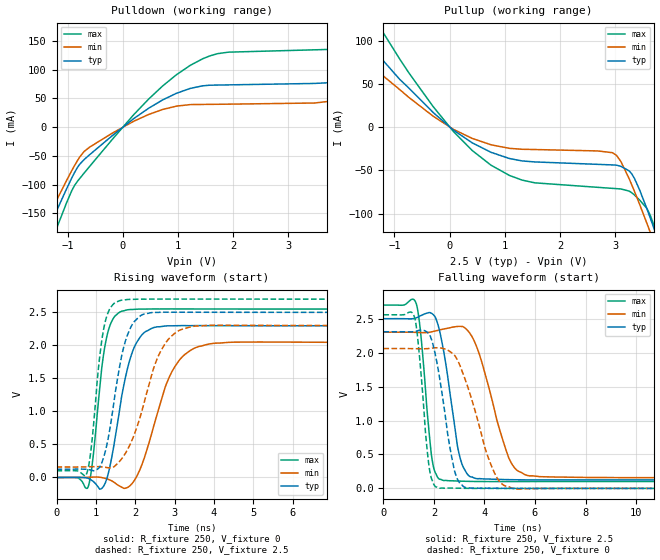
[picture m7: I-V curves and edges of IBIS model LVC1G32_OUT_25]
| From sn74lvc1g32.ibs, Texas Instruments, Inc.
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[Model]   LVC1G32_OUT_25
Model_type  Output
Vref =   0.0
Rref =   500
Cref =   30p
Vmeas =   1.25
| variable   typ   min   max
C_comp   7.81pF   3.37pF   14.37pF
| C_pullup   6.28pF   3.37pF   8.33pF
| C_pulldown   9.34pF   4.59pF   14.37pF
[Temperature Range]   40   100   -40
| Ambient temperature   25   85   -40
[Voltage range]   2.5   2.3   2.7
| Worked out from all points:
|   slope of the pulldown table from 0 to 0.375 V, typ, clamps not added: 13.9 ohm
|   slope of the pullup table from 0 to 0.375 V, typ, clamps not added: 22 ohm
|   rising waveform, R_fixture 250, V_fixture 0: 20-80 % time 442ps typ, 674ps min, 282ps max; typ from 0 V to 2.3 V
|   rising waveform, R_fixture 250, V_fixture 2.5: 20-80 % time 416ps typ, 679ps min, 265ps max; typ from 0.125 V to 2.5 V
|   falling waveform, R_fixture 250, V_fixture 2.5: 20-80 % time 561ps typ, 950ps min, 361ps max; typ from 2.5 V to 0.125 V
|   falling waveform, R_fixture 250, V_fixture 0: 20-80 % time 581ps typ, 997ps min, 347ps max; typ from 2.31 V to 0 V
[Pulldown]
| LVC1G32_OUT_25
|   Voltage   I(typ)   I(min)   I(max)
-5V       -964.5mA   -872.8mA   -1.115A
-1.565V   -226.1mA   -199.4mA   -269.6mA
-1.175V   -140.9mA   -122.9mA   -170.6mA
-700mV    -56.58mA   -42.46mA   -80.14mA
-200mV    -15.69mA   -11.1mA    -22.59mA
725mV     47.53mA    30.83mA    71.89mA
1.715V    73.33mA    39.84mA    128mA
3.965V    81.26mA    49.43mA    136.9mA
5.285V    134.2mA    90.34mA    197.6mA
5.95V     167mA      44.61mA    249.8mA
6.55V     83.02mA    45.06mA    295.2mA
10V       87.5mA     48.06mA    154.1mA
[Pullup]
| LVC1G32_OUT_25
|   Voltage   I(typ)   I(min)   I(max)
-5V       437mA      352.6mA    602.5mA
-2.275V   165.5mA    130.1mA    232.1mA
-1.71V    117mA      91.04mA    165mA
-1.21V    77.47mA    59.63mA    110mA
-300mV    17.08mA    12.74mA    23.93mA
750mV     -29.15mA   -20.41mA   -44.03mA
1.545V    -40.27mA   -25.92mA   -64.48mA
2.95V     -43.75mA   -29.57mA   -70.87mA
3.3V      -53.93mA   -66.55mA   -75.91mA
3.635V    -104.8mA   -121.4mA   -101.8mA
3.725V    -121mA     -136.9mA   -117.4mA
10V       -1.408A    -1.338A    -1.542A
[Ramp]
| LVC1G32_OUT_25
| variable   typ   min   max
dV/dt_r   1.49/4.74E-10   1.33/7.46E-10   1.63/3.00E-10
dV/dt_f   1.48/5.92E-10   1.34/1.04E-09   1.61/3.84E-10
R_load = 250
[Rising Waveform]
| LVC1G32_OUT_25
R_fixture =   250
C_fixture =   0
L_fixture =   0
V_fixture =   0
V_fixture_min = 0
V_fixture_max = 0
|   Time   V(typ)   V(min)   V(max)
0s        -58.09uV   -70.55uV   -30.79uV
805ps     -13.61mV   2.943mV    -139.6mV
925ps     -56.35mV   5.269mV    288.7mV
1.195ns   -133.2mV   -7.064mV   1.86V
1.435ns   407.5mV    -62.26mV   2.401V
1.85ns    1.755V     -133.2mV   2.542V
2.23ns    2.196V     294.9mV    2.549V
2.98ns    2.296V     1.652V     2.551V
4.035ns   2.298V     2.033V     2.551V
50ns      2.296V     2.045V     2.55V
[Rising Waveform]
| LVC1G32_OUT_25
R_fixture =   250
C_fixture =   0
L_fixture =   0
V_fixture =   2.5
V_fixture_min = 2.3
V_fixture_max = 2.7
|   Time   V(typ)   V(min)   V(max)
0s        125.2mV    158.6mV    101.1mV
770ps     123.5mV    160.9mV    64.97mV
890ps     109.6mV    162.8mV    492.1mV
1.105ns   164.7mV    162.4mV    1.869V
1.345ns   699.1mV    145.4mV    2.544V
1.63ns    1.764V     263.9mV    2.681V
1.815ns   2.175V     434.8mV    2.695V
2.66ns    2.502V     1.927V     2.701V
3.56ns    2.502V     2.294V     2.701V
50ns      2.5V       2.3V       2.7V
[Falling Waveform]
| LVC1G32_OUT_25
R_fixture =   250
C_fixture =   0
L_fixture =   0
V_fixture =   2.5
V_fixture_min = 2.3
V_fixture_max = 2.7
|   Time   V(typ)   V(min)   V(max)
0s        2.5V       2.3V       2.7V
1.305ns   2.512V     2.298V     2.716V
1.92ns    2.575V     2.307V     443.2mV
2.38ns    2.03V      2.347V     116.6mV
2.93ns    623.8mV    2.385V     108.5mV
3.3ns     222mV      2.339V     104.2mV
3.81ns    144.2mV    1.961V     101.2mV
4.965ns   129mV      445.4mV    100.5mV
5.775ns   125.3mV    184.4mV    100.7mV
50ns      125.2mV    158.6mV    101.1mV
[Falling Waveform]
| LVC1G32_OUT_25
R_fixture =   250
C_fixture =   0
L_fixture =   0
V_fixture =   0
V_fixture_min = 0
V_fixture_max = 0
|   Time   V(typ)   V(min)   V(max)
0s        2.307V     2.059V     2.557V
1.235ns   2.309V     2.058V     2.516V
1.375ns   2.325V     2.057V     2.148V
1.805ns   2.276V     2.061V     327.3mV
2.225ns   1.626V     2.071V     2.616mV
2.675ns   516.5mV    2.005V     4.479mV
2.99ns    93.65mV    1.844V     2.815mV
4.375ns   2.068mV    245.5mV    -529.4uV
5.255ns   -2.195uV   -9.901mV   -306.4uV
50ns      -47.81uV   -51uV      -17.66uV
